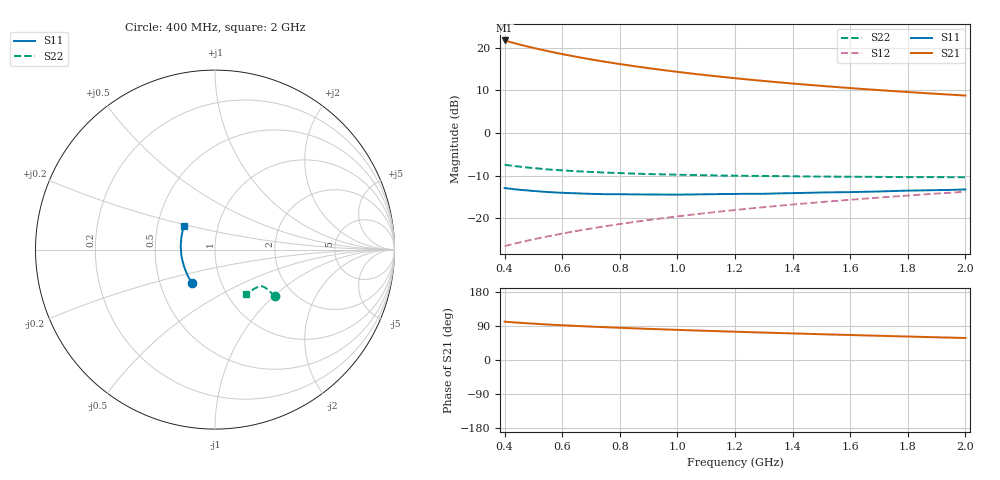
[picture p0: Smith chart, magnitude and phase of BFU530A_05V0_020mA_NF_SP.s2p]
! Filename:  P:\Prog\Test\Noise\ATS_data\Testdata_Net\06 Compressed Noise after Statistics\BFU530A_APG2013_33_A05_05p0V_020mA_NF_CM01_D.sf
! Date/Time: Tue 16/Apr/2013 15:10:57
! BFU530A_APG2013_33_A05_05p0V_1to25mA_NF_CM01_Bias7_R.sf
! Noise Parameter Data File
! BFU530A_APG2013_33_A05_05p0V_1to25mA_NF_CM01
! Date/time: Fri Apr 12 15:27:54 2013
! VAR V_out= 5.001000
! VAR I_out= 20.000000
! VAR V_in= 0.839000
! VAR I_in= 0.218150
! Device data file deembeded for feedlines and parallel
! Original file: \06 Compressed Noise after Statistics\BFU530A_APG2013_33_A05_05p0V_020mA_NF_CM01_R.sf
! Feed-files: PR017V01_150413_Feed1.s2p, PR017V01_150413_Feed2.s2p
! Parallel-file: PR017V01_150413_Par.s2p
# MHz S MA R 50
!  Freq-MHz  S11-mag  S11-arg  S21-mag  S21-arg  S12-mag  S12-arg  S22-mag  S22-arg
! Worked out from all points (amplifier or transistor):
!   37 points, 400 MHz to 2 GHz, reference 50 ohm
!   highest |S21| = 21.7 dB at 400 MHz (marker M1)
!   |S21| within 3 dB of that: start of sweep to 585.7 MHz
!   unconditionally stable (mu >= 1): 972.8 MHz to 1.957 GHz
!   at 500 MHz: K = 0.93, MSG = 22.5 dB, |S12| = -25.0 dB
!   at 1.1 GHz: K = 1.00, MAG = 15.8 dB, |S12| = -18.8 dB
!   at 2 GHz: K = 1.00, MSG = 11.3 dB, |S12| = -13.8 dB
!   lowest NFmin = 1.01 dB at 420 MHz
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400  0.2255 -124.6  12.18 101.1  0.04696 71.4  0.4234 -37.8
420  0.2216 -127.3  11.66 99.9  0.04888 71.6  0.4145 -37.7
440  0.2178 -130.1  11.18 98.8  0.05075 71.8  0.4069 -37.6
480  0.2117 -135.1  10.33 96.8  0.05455 72.1  0.3931 -37.5
500  0.2086 -137.4  9.955 95.9  0.05647 72.2  0.3875 -37.5
550  0.2026 -143.1  9.137 93.6  0.06116 72.6  0.3734 -37.2
600  0.1985 -148.0  8.424 91.7  0.066 72.8  0.3639 -37.1
650  0.1957 -152.5  7.821 89.9  0.07085 72.9  0.3558 -37.2
700  0.193 -156.7  7.297 88.1  0.07566 73.0  0.3489 -37.2
750  0.1913 -160.7  6.838 86.5  0.08054 73.1  0.3428 -37.4
800  0.191 -164.2  6.437 85.0  0.08541 73.1  0.3382 -37.6
850  0.1901 -168.0  6.08 83.5  0.09027 73.1  0.3333 -38.0
900  0.1898 -171.3  5.76 82.2  0.09518 73.0  0.3295 -38.3
950  0.1894 -174.3  5.473 80.8  0.1001 72.9  0.3266 -38.7
1050  0.1898 179.9  4.979 78.2  0.1099 72.6  0.3214 -39.6
1100  0.1908 177.4  4.766 77.0  0.1149 72.4  0.3193 -40.1
1200  0.1926 172.3  4.392 74.7  0.1248 72.0  0.3155 -41.4
1350  0.1953 165.4  3.934 71.2  0.1396 71.2  0.3116 -43.4
1500  0.2004 159.2  3.569 68.0  0.1545 70.3  0.3076 -45.7
1650  0.2043 153.8  3.271 64.9  0.1695 69.3  0.3059 -48.3
1750  0.2084 150.4  3.1 62.9  0.1794 68.6  0.3042 -50.0
2000  0.2176 142.7  2.75 58.1  0.2042 66.7  0.3024 -54.9
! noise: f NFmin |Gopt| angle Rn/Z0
400  1.068  0.2413  -168.9  0.0842
460  1.061  0.2545  -166.7  0.0774
600  1.082  0.2577  -160.1  0.0961
800  1.101  0.2852  -158.9  0.0776
1000  1.128  0.3018  -153.5  0.0784
1200  1.161  0.306  -146.9  0.0872
1400  1.176  0.3123  -143  0.0953
1600  1.185  0.342  -136.6  0.099
1800  1.194  0.3579  -132.4  0.1036
2000  1.201  0.3783  -128  0.1129
